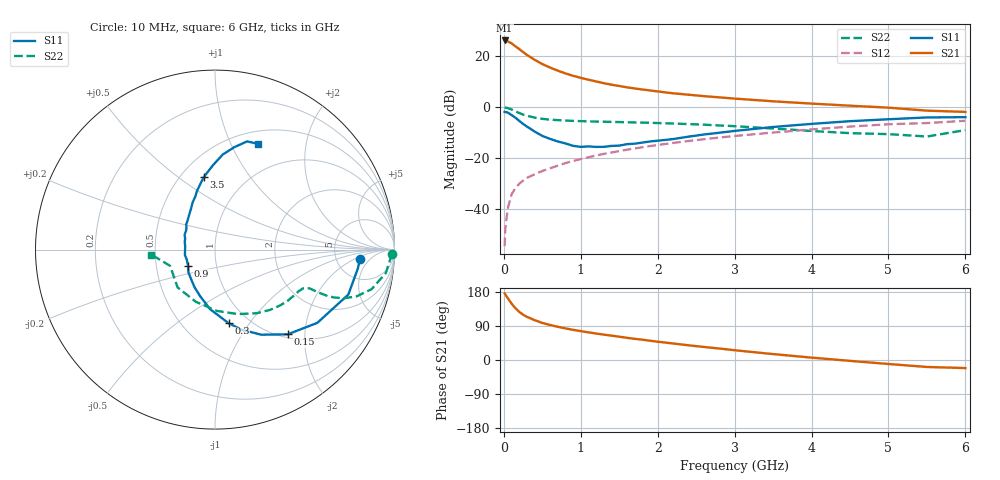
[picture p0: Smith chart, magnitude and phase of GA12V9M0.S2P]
! Infineon Technologies  Discrete & RF Semiconductors
! BF775
! Si NPN RF Bipolar Junction Transistor in SOT23
! VCE = 12 V  IC = 9 mA
! Common Emitter S-Parameters:  May  1996
# GHz  S  MA  R  50
!  f  S11  S21  S12  S22
! GHz  MAG  ANG  MAG  ANG  MAG  ANG  MAG  ANG
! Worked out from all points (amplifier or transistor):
!   36 points, 10 MHz to 6 GHz, reference 50 ohm
!   highest |S21| = 26.1 dB at 10 MHz (marker M1)
!   |S21| within 3 dB of that: start of sweep to 183.4 MHz
!   unconditionally stable (mu >= 1): 683.1 MHz to 2.74 GHz
!   at 250 MHz: K = 0.62, MSG = 25.2 dB, |S12| = -28.8 dB
!   at 1.4 GHz: K = 1.09, MAG = 11.4 dB, |S12| = -17.8 dB
!   at 6 GHz: K = 0.86, MSG = 1.7 dB, |S12| = -5.3 dB
!   S11 on the Smith chart (normalised r, x): 10 MHz: 8.66, -2.61; 150 MHz: 1.06, -1.64; 300 MHz: 0.81, -0.80; 900 MHz: 0.73, -0.13; 3.5 GHz: 0.64, +0.63; 6 GHz: 0.64, +1.27
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0.01  0.8087 -3.7  20.2 175.9  0.0019 86.5  0.9881 -1.5
0.02  0.8032 -7.4  19.73 172.6  0.0043 81.3  0.9779 -3.2
0.05  0.784 -18.6  19.37 163.4  0.0102 78.4  0.9607 -7.8
0.1  0.7012 -35.6  17.77 149.0  0.0195 72.5  0.8998 -14.2
0.15  0.6218 -49.4  15.54 136.7  0.0261 68.1  0.8303 -18.3
0.2  0.5395 -61.5  13.72 127.1  0.0315 64.8  0.7672 -20.7
0.25  0.4691 -71.8  11.99 119.6  0.0365 62.4  0.7149 -21.9
0.3  0.4171 -79.5  10.53 113.9  0.0412 62.4  0.6779 -22.4
0.4  0.3331 -94.7  8.455 105.2  0.0485 62.5  0.6251 -22.5
0.5  0.2735 -107.4  6.972 97.8  0.0561 63.5  0.5901 -22.4
0.6  0.2393 -118.3  5.955 92.5  0.0636 64.0  0.5698 -22.3
0.7  0.2131 -128.3  5.186 87.7  0.0716 64.8  0.5572 -22.6
0.9  0.1748 -149.3  4.11 79.6  0.0882 65.1  0.5382 -23.6
1.1  0.1703 -170.0  3.442 73.0  0.1046 65.2  0.5267 -25.4
1.3  0.167 173.9  2.943 67.0  0.1217 64.6  0.5179 -27.3
1.6  0.1886 153.9  2.444 58.5  0.1468 63.2  0.5058 -31.2
2.2  0.2372 127.9  1.867 43.6  0.1993 59.3  0.4784 -40.4
2.6  0.2913 115.3  1.641 34.4  0.2353 55.9  0.4539 -47.9
3.5  0.409 98.8  1.301 15.6  0.3182 46.8  0.3814 -70.4
4.5  0.5309 85.4  1.068 -2.3  0.4165 35.1  0.3097 -110.2
5.5  0.6286 73.5  0.854 -18.4  0.488 19.9  0.266 -160.1
6  0.6365 67.9  0.807 -21.3  0.5407 15.7  0.3555 -175.5
